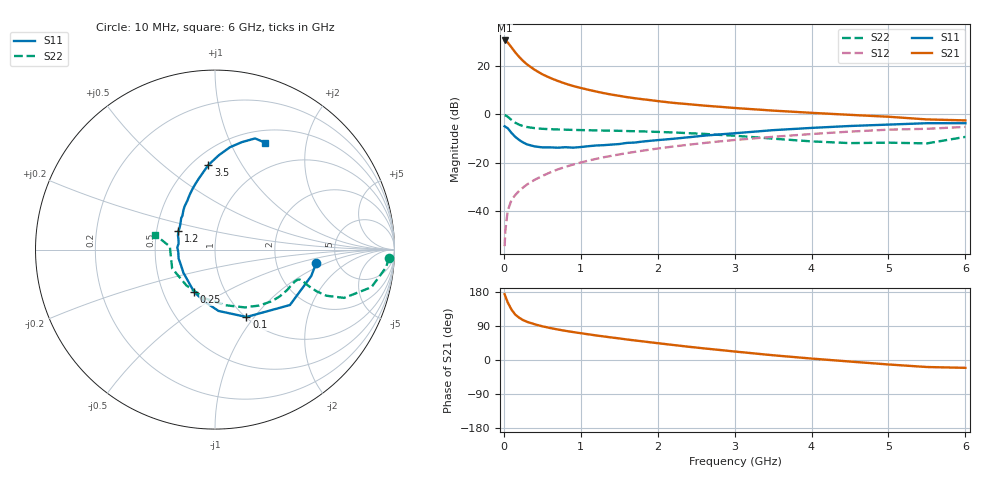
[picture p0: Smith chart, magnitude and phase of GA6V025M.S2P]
! Infineon Technologies  Discrete & RF Semiconductors
! BF775
! Si NPN RF Bipolar Junction Transistor in SOT23
! VCE = 6 V  IC = 25 mA
! Common Emitter S-Parameters:  May  1996
# GHz  S  MA  R  50
!  f  S11  S21  S12  S22
! GHz  MAG  ANG  MAG  ANG  MAG  ANG  MAG  ANG
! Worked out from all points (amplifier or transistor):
!   36 points, 10 MHz to 6 GHz, reference 50 ohm
!   highest |S21| = 30.5 dB at 10 MHz (marker M1)
!   |S21| within 3 dB of that: start of sweep to 103 MHz
!   unconditionally stable (mu >= 1): 371.6 MHz to 2.681 GHz
!   at 250 MHz: K = 0.89, MSG = 26.1 dB, |S12| = -30.2 dB
!   at 1.4 GHz: K = 1.11, MAG = 10.6 dB, |S12| = -17.1 dB
!   at 6 GHz: K = 0.92, MSG = 1.3 dB, |S12| = -5.2 dB
!   S11 on the Smith chart (normalised r, x): 10 MHz: 3.44, -0.78; 100 MHz: 1.01, -0.91; 250 MHz: 0.72, -0.37; 1.2 GHz: 0.65, +0.14; 3.5 GHz: 0.60, +0.73; 6 GHz: 0.65, +1.36
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0.01  0.5685 -7.8  33.67 173.7  0.0019 86.4  0.9708 -2.6
0.02  0.5559 -15.4  33.17 167.9  0.004 81.3  0.9584 -5.9
0.05  0.5193 -36.5  30.57 152.2  0.0102 75.6  0.8965 -13.5
0.1  0.4142 -65.0  24.18 132.8  0.0172 68.7  0.7684 -20.5
0.15  0.3423 -86.7  18.98 119.5  0.0218 66.6  0.6715 -22.5
0.2  0.296 -101.2  15.34 111.4  0.0264 66.9  0.6119 -22.3
0.25  0.2638 -115.9  12.71 105.3  0.0309 67.4  0.574 -21.6
0.3  0.2408 -124.9  10.84 100.8  0.0356 69.5  0.5492 -20.9
0.4  0.2183 -143.7  8.362 94.4  0.0446 70.4  0.5212 -19.8
0.5  0.2083 -156.3  6.748 88.9  0.0535 71.6  0.5041 -19.5
0.6  0.2087 -166.5  5.691 84.5  0.0631 71.9  0.4948 -19.7
0.7  0.2051 -176.0  4.922 80.5  0.0731 72.0  0.4886 -20.2
0.8  0.2102 176.9  4.322 77.0  0.0824 71.4  0.4833 -21.1
0.9  0.2056 170.5  3.864 73.7  0.092 71.1  0.4783 -21.9
1.1  0.2206 159.1  3.222 67.8  0.1111 70.0  0.4711 -24.6
1.2  0.2282 153.6  2.972 64.8  0.1208 69.4  0.4672 -25.8
1.6  0.258 136.8  2.275 54.1  0.159 65.9  0.4529 -31.9
2.2  0.3135 119.4  1.734 39.7  0.2169 60.3  0.4243 -43.1
3.5  0.4728 94.5  1.198 12.5  0.3444 45.2  0.3157 -79.2
4.5  0.5764 81.7  0.979 -4.1  0.4417 31.9  0.2554 -128.5
5.5  0.6583 70.2  0.788 -18.5  0.5047 16.2  0.252 176.1
6  0.6578 65.1  0.752 -20.7  0.5517 11.9  0.3435 166.1
